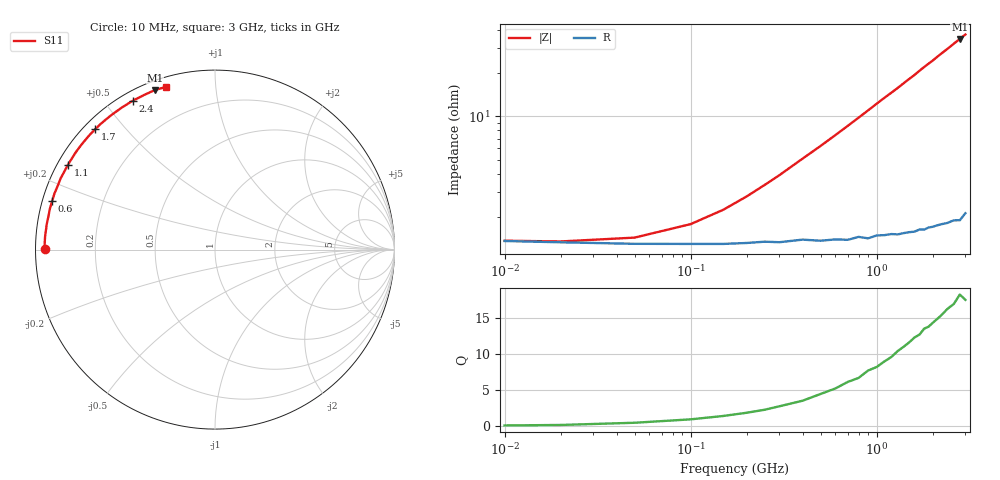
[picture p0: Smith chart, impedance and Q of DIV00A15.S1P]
! SIEMENS Small Signal Semiconductors
! BAV99
! Silicon Switching Diode in SOT23
! IF = 150 mA
! S-Parameters:  May  1995
# GHz  S  MA  R  50
!  f  S11
! GHz  MAG  ANG
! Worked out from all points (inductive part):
!   30 points, 10 MHz to 3 GHz, reference 50 ohm
!   read as one part to ground: L = 1.94 nH near 400 MHz
!   highest Q = 17.5 at 2.8 GHz (marker M1), where L = 1.97 nH
!   S11 on the Smith chart (normalised r, x): 10 MHz: 0.03, +0.00; 600 MHz: 0.03, +0.15; 1.1 GHz: 0.03, +0.27; 1.7 GHz: 0.03, +0.41; 2.4 GHz: 0.04, +0.59; 3 GHz: 0.04, +0.74
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0.01  0.947 179.7
0.02  0.9481 179.5
0.05  0.9493 178.6
0.15  0.9495 175.8
0.25  0.9478 173.0
0.3  0.9483 171.6
0.4  0.9464 168.8
0.5  0.9476 166.1
0.6  0.9468 163.4
0.7  0.9475 160.7
0.8  0.9455 158.0
0.9  0.9473 155.3
1  0.9454 152.6
1.1  0.9458 150.0
1.2  0.9455 147.5
1.3  0.9465 145.0
1.4  0.9462 142.4
1.5  0.9462 139.9
1.6  0.9466 137.5
1.7  0.9457 134.9
1.8  0.9468 132.4
1.9  0.946 130.1
2  0.9463 127.9
2.2  0.9466 123.2
2.4  0.9475 118.9
2.6  0.9477 114.6
2.8  0.95 110.6
3  0.9468 106.7
